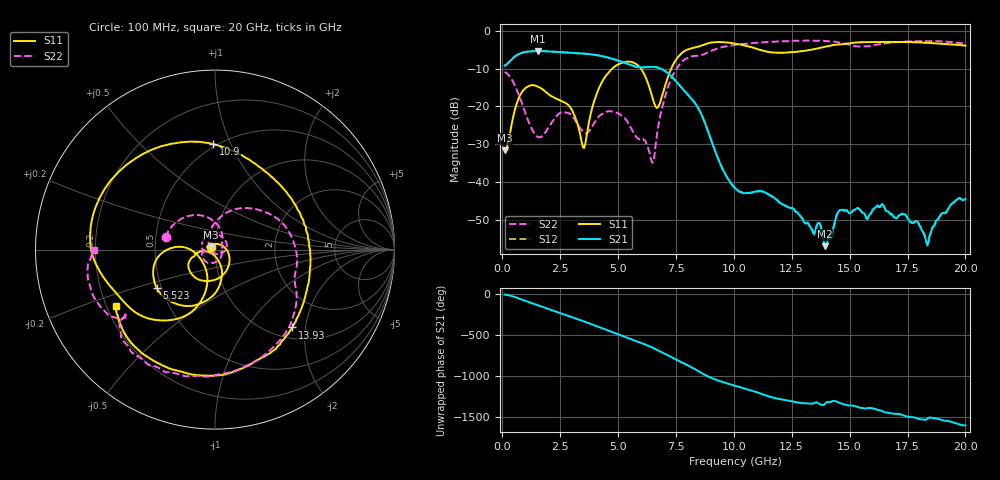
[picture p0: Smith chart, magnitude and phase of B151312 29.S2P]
!  2-Port S-parameters saved by WinCal
! VAR MeasName=S-Parameters (CALIBRATED_DATA) read from VNA (N5244A)
! VAR MeasDate=12/8/2015 5:45:42 PM
! VAR NAME=B151312 29
! VAR FILENAME=B151312 29.S2P
! VAR DATE=12/8/2015 5:45:42 PM
! VAR PHYS_PORTS=1,2
# Hz S DB R 50
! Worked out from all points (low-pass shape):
!   401 points, 100 MHz to 20 GHz, reference 50 ohm
!   highest |S21| = -5.41 dB at 1.543 GHz (marker M1); lowest = -56.8 dB at 13.93 GHz (marker M2)
!   |S21| within 3 dB of the highest: 272.2 MHz to 5.244 GHz (4.971 GHz wide, 180 % of centre)
!   lowest |S11| = -31.5 dB at 100 MHz (marker M3), VSWR 1.05, Z = 47.7 + j1.2 ohm
!   |S11| at or under -10 dB: start of sweep to 4.756 GHz; 5.984 GHz to 7.298 GHz (1.315 GHz wide, 19.8 % of centre)
!   |S22| runs from -34.8 to -2.6 dB; largest |S21 - S12| = 0.0015
!   S11 on the Smith chart (normalised r, x): 100 MHz: 0.95, +0.02; 5.523 GHz: 0.47, -0.24; 10.9 GHz: 0.48, +0.86; 13.93 GHz: 1.22, -1.70; 20 GHz: 0.24, -0.25
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1e8  -31.53 151.6  -9.25 -4.2  -9.24 -4.2  -10.94 166.1
7.965e8  -16.76 -70.7  -5.98 -60.0  -5.97 -60.0  -18.23 77.4
1.54275e9  -14.79 -142.0  -5.41 -135.7  -5.40 -135.8  -27.99 14.0
2.09e9  -17.16 -160.7  -5.51 170.6  -5.51 170.6  -24.69 -64.6
2.63725e9  -18.79 -165.3  -5.72 117.3  -5.72 117.3  -21.44 -127.8
3.43325e9  -29.51 -150.9  -6.03 38.3  -6.02 38.3  -26.18 -179.0
3.93075e9  -19.31 -70.6  -6.33 -13.2  -6.33 -13.2  -24.80 -170.6
4.52775e9  -11.52 -94.5  -7.04 -76.8  -7.04 -76.8  -21.39 130.4
5.52275e9  -8.21 -146.9  -9.01 176.7  -9.01 176.6  -25.34 -9.9
6.468e9  -17.33 -179.8  -9.55 72.1  -9.54 72.0  -34.78 -123.0
6.7665e9  -19.72 -127.3  -9.84 30.8  -9.84 30.8  -24.20 127.1
7.7615e9  -5.87 -129.4  -15.19 -111.3  -15.14 -111.5  -8.18 25.8
9.00525e9  -3.18 178.6  -28.62 64.1  -28.63 63.6  -5.39 -32.6
1.005e10  -3.42 131.3  -41.47 -33.6  -41.51 -33.9  -3.77 -64.4
1.089575e10  -4.62 90.9  -42.43 -103.6  -42.56 -103.9  -3.23 -83.2
1.228875e10  -5.76 23.6  -46.40 149.4  -46.39 148.8  -2.82 -107.1
1.338325e10  -5.01 -25.7  -52.58 108.7  -52.38 109.4  -2.68 -123.0
1.39305e10  -4.27 -45.1  -56.80 106.9  -56.82 110.1  -2.74 -130.6
1.457725e10  -3.66 -67.0  -47.28 115.7  -47.22 116.3  -3.20 -139.7
1.67165e10  -3.01 -113.6  -47.98 -6.8  -47.78 -6.3  -3.19 -147.5
1.835825e10  -3.25 -136.0  -56.65 -74.2  -56.33 -73.6  -2.79 -164.1
2e10  -3.96 -150.3  -44.34 -156.8  -44.44 -158.6  -3.41 -179.7
